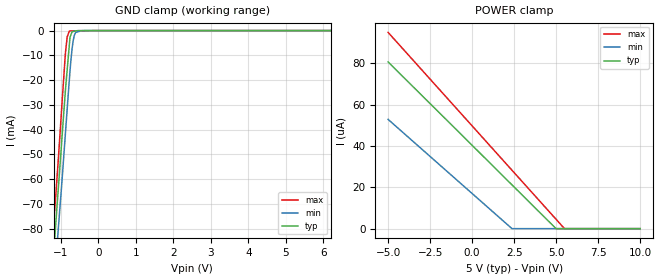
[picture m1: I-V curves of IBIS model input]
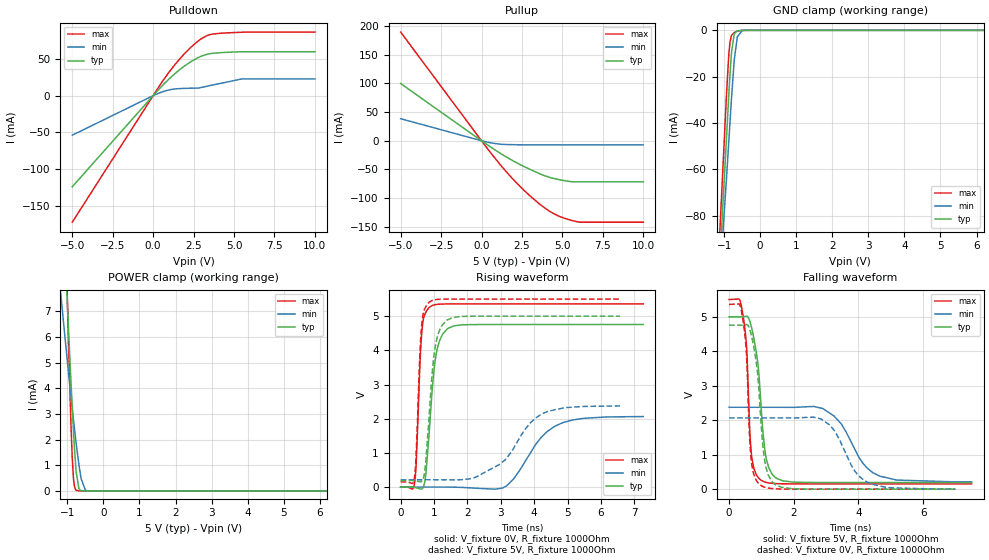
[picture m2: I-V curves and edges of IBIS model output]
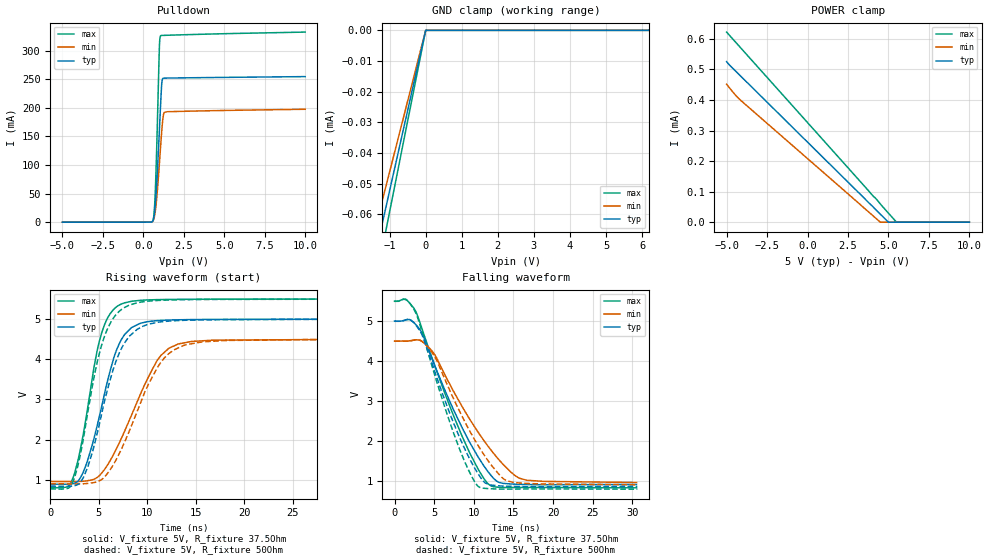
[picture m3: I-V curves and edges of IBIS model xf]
|Texas Instruments Incorporated
| ControlNet(TM) Transceiver
| Marketing part#   Digital Voltage Range   Package-type   #pins
| SN65HVD61D   2.375V-5.5V   SOIC   14
| SN65HVD61DG4   2.375V-5.5V   SOIC   14
| SN65HVD61DR   2.375V-5.5V   SOIC   14
| SN65HVD61DRG4   2.375V-5.5V   SOIC   14
[IBIS Ver]   4.1
[File name]   sn65hvd61.ibs
[File Rev]   1.0
[Date]   6/26/2013
[Source]
| Texas Instruments Incorporated.
| Analog-eLab Design Center, HPA
| 12500 TI Blvd
| Dallas, TX -75243
[Notes]   Revision History:
| Rev 1.0: 6/26/2013
| - Initial version of the model
| - Model generated from simulations in TISPICE
| - Model matched to SPICE simulation
| - C_comp although listed in numerical order of value are
|   obtained from varying PVT conditions. For PVT conditions for
|   each specific value refer the buffer description under
|   respective [Model]. IBIS model user is responsible for using
|   appropriate C_comp to simulate for Signal Integrity.
|*  EXCEPTION   *
|*  - For model input,There will be a leakage current in the power clamp I-V  *
|*   Table because of the pulldown R2(RES_P1H) resistance connected between  *
|*   ground and pad pin .   *
|*  - For model xf,There will be a leakage current in the power clamp I-V   *
|*   Table because of the RES_P1H resistances connected between   *
|*   ground and pad pin from the attenuation block   *
[Disclaimer]
| This model is designed as an aid for customers of Texas Instruments.
| TI and its licensors and suppliers make no warranties, either expressed
| or implied, with respect to this  model, including the warranties of
| merchantability or fitness for a particular purpose. The model is
| provided solely on an "as is" basis. The entire risk as to its quality
| and performance is with the customer.
[Copyright]
(C) Copyright 2013 Texas Instruments Incorporated.All rights reserved.
|   SN65HVD61
[Component]   SN65HVD61
[Manufacturer]   TI
[Package]   |14 SOIC  -  D package
|   typ   min   max
R_pkg   0.1052025   0.05633   0.14242
L_pkg   2.5378625nH  1.72746nH   3.46735nH
C_pkg   0.462875pF   0.35056pF   0.62881pF
[Pin]  signal_name   model_name   R_pin   L_pin   C_pin
1   RX   output   0.11216   3.36701nH  0.62881pF
2   CD   output   0.14102   2.79716nH  0.46799pF
3   VDD   power   0.06385   1.94248nH  0.40989pF
4   CHEN   input   0.09802   2.01847nH  0.35056pF
5   TX   input   0.11457   2.26018nH  0.36209pF
6   _TX   input   0.14242   2.82725nH  0.46580pF
7   TXEN   input   0.11690   3.46735nH  0.62224pF
8   SIG   nc   0.11238   3.40402nH  0.62049pF
9   DGND   gnd   0.06099   2.01080nH  0.49310pF
10   XF3   xf   0.06020   1.83802nH  0.40525pF
11   CGND   gnd   0.05087   1.61450nH  0.38992pF
12   XF1   xf   0.05633   1.72746nH  0.40026pF
13   CGND   gnd   0.06099   2.02284nH  0.49854pF
14   VCC   power   0.05843   3.02226nH  0.66420pF
| Models and submodels in the file (3): input (Input), output (3-state), xf (I/O_open_sink)
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|   input Model
[Model]   input
Model_type   Input
Vinl = 1.5
Vinh = 3.5
|   typ   min   max
|   (nom PVT)   (fast PVT)   (slow PVT)
C_comp   1.465e-12   1.413e-12   1.777e-12
[Model spec]
|subparameter
Vinl   1.5   0.7125   1.65
Vinh   3.50   1.6625   3.85
| Where nom  PVT is Nominal Process, 5V, 27C
|   Fast PVT is Strong Process,  5.5V, -30C
|   Slow PVT is Weak Process,   2.375V, 100C
[Voltage Range]   5   2.375   5.5
|Junction Temperature
[Temperature Range]   27   100   -30
[Power Clamp Reference]   5   2.375   5.5
[GND Clamp Reference]   0   0   0
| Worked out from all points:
|   GND clamp passes 1 mA (typ) near -0.72 V on its own axis
[GND Clamp]
|   Voltage   I(typ)   I(min)   I(max)
-5V       -570.9mA   -618.4mA   -543.7mA
-1.223V   -95.42mA   -107.8mA   -83.36mA
-1.171V   -84.48mA   -98.48mA   -72.9mA
-1.144V   -78.85mA   -93.5mA    -67.51mA
-1.081V   -65.58mA   -81.73mA   -53.82mA
-880mV    -23.57mA   -41.01mA   -8.722mA
-836mV    -15.92mA   -31.8mA    -2.607mA
-764.5mV  -3.497mA   -17.24mA   -153.8uA
-707.7mV  -549.9uA   -7.753mA   -142.4uA
-646mV    -261.4uA   -2.023mA   -129.9uA
-439.4mV  -4.594uA   -7.683uA   -88.38uA
10V       0A         0A         0A
[POWER Clamp]
|   Voltage   I(typ)   I(min)   I(max)
-5V       80.61uA    52.82uA    94.88uA
2.373V    21.18uA    17.01nA    28.26uA
4.995V    40.31nA    0A         4.563uA
5.495V    0A         0A         49.7nA
10V       0A         0A         0A
|   output Model
[Model]   output
Model_type   3-state
Polarity   Non-Inverting
Vmeas = 2.0
Vref = 0
Cref = 15pF
Rref = 1000
|   typ   min   max
|   (nom PVT)   (fast PVT)   (slow PVT)
C_comp   2.533e-12   2.400e-12   3.277e-12
| Where nom  PVT is Nominal Process, 5V, 27C
|   Fast PVT is Strong Process,  5.5V, -30C
|   Slow PVT is Weak Process,   2.375V, 100C
[Voltage Range]   5   2.375   5.5
|Junction Temperature
[Temperature Range]   27   100   -30
[Pullup Reference]   5   2.375   5.5
[Pulldown Reference]   0   0   0
[Power Clamp Reference]   5   2.375   5.5
[GND Clamp Reference]   0   0   0
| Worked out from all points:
|   slope of the pulldown table from 0 to 0.75 V, typ, clamps not added: 42.3 ohm
|   slope of the pullup table from 0 to 0.75 V, typ, clamps not added: 52.3 ohm
|   GND clamp passes 1 mA (typ) near -0.69 V on its own axis
|   POWER clamp passes 1 mA (typ) near -0.77 V on its own axis
|   falling waveform, V_fixture 5V, R_fixture 1000Ohm: 20-80 % time 275ps typ, 816ps min, 157ps max; typ from 5 V to 0.193 V
|   rising waveform, V_fixture 0V, R_fixture 1000Ohm: 20-80 % time 249ps typ, 920ps min, 134ps max; typ from 0 V to 4.76 V
|   rising waveform, V_fixture 5V, R_fixture 1000Ohm: 20-80 % time 242ps typ, 1.02ns min, 131ps max; typ from 0.193 V to 5 V
|   falling waveform, V_fixture 0V, R_fixture 1000Ohm: 20-80 % time 263ps typ, 697ps min, 154ps max; typ from 4.76 V to 0 V
[Pulldown]
|   Voltage   I(typ)   I(min)   I(max)
-5V       -124.3mA   -53.93mA   -172.6mA
0V        0A         0A         0A
557.5mV   13.43mA    5.13mA     18.87mA
989.8mV   22.89mA    7.871mA    32.21mA
1.617V    35.01mA    9.62mA     49.47mA
2.004V    41.48mA    9.97mA     58.84mA
2.75V     51.51mA    10.34mA    73.89mA
3.404V    56.8mA     13.24mA    82.5mA
4.202V    58.74mA    16.92mA    85.2mA
5.502V    59.92mA    22.88mA    86.51mA
10V       59.92mA    22.88mA    86.72mA
[GND Clamp]
|   Voltage   I(typ)   I(min)   I(max)
-5V       -869.5mA   -740.6mA   -996mA
-1.145V   -107.2mA   -113.8mA   -95.34mA
-935.5mV  -47.05mA   -64.31mA   -28.26mA
-875mV    -29.39mA   -49.25mA   -11.67mA
-865mV    -26.58mA   -46.74mA   -9.576mA
-836.5mV  -18.97mA   -39.62mA   -5.105mA
-792.5mV  -9.229mA   -28.85mA   -2.14mA
-715mV    -1.413mA   -12.29mA   -929.1uA
-632.4mV  -210.3uA   -2.765mA   -373uA
-500mV    -7.452uA   -137.4uA   -26.2uA
-375.9mV  -165.6nA   -7.725uA   -510.1nA
10V       0A         0A         0A
[Pullup]
|   Voltage   I(typ)   I(min)   I(max)
-5V       99.82mA    38.45mA    189.5mA
0V        0A         0A         0A
697.6mV   -13.38mA   -4.226mA   -25.64mA
1.605V    -29.37mA   -6.596mA   -56.31mA
2.381V    -41.42mA   -6.991mA   -79.63mA
3.692V    -58.6mA    -7.139mA   -112.5mA
4.29V     -64.44mA   -7.139mA   -124.3mA
4.806V    -67.79mA   -7.139mA   -131.7mA
5.5V      -71.17mA   -7.139mA   -138.3mA
6.061V    -71.58mA   -7.139mA   -141.9mA
10V       -71.58mA   -7.139mA   -141.9mA
[POWER Clamp]
|   Voltage   I(typ)   I(min)   I(max)
-5V       144.5mA    65.18mA    243.7mA
-1.315V   17.65mA    9.659mA    25.67mA
-1.15V    12.15mA    7.204mA    15.93mA
-1.008V   7.54mA     5.164mA    7.89mA
-902.5mV  4.327mA    3.722mA    2.689mA
-864mV    3.232mA    3.213mA    1.27mA
-805mV    1.721mA    2.457mA    187.1uA
-754mV    718.4uA    1.836mA    22.06uA
-680mV    82.57uA    1.021mA    1.038uA
-618.1mV  8.277uA    474.2uA    87.89nA
-442.4mV  0A         5.444uA    0A
10V       0A         0A         0A
[Ramp]
R_load = 1000
|   typ   min   max
dV/dt_r   2.85414/2.46472e-10   1.23967/9.10375e-10   3.21465/1.33896e-10
dV/dt_f   2.88408/2.73849e-10   1.29658/8.04689e-10   3.20839/1.56294e-10
[Falling Waveform]
V_fixture = 5V
V_fixture_min = 2.375V
V_fixture_max = 5.5V
R_fixture = 1000Ohm
|   Time   V(typ)   V(min)   V(max)
0s        5V         2.375V     5.5V
432ps     4.998V     2.375V     5.048V
544ps     5.019V     2.375V     4.099V
688ps     4.721V     2.375V     1.06V
970ps     2.707V     2.375V     275mV
1.156ns   864.2mV    2.375V     194.9mV
1.65ns    244.4mV    2.374V     155.6mV
3.248ns   193.2mV    2.12V      152.7mV
4.652ns   193.2mV    378.9mV    152.7mV
7.5ns     193.2mV    214mV      152.7mV
[Rising Waveform]
V_fixture = 0V
V_fixture_min = 0V
V_fixture_max = 0V
R_fixture = 1000Ohm
|   Time   V(typ)   V(min)   V(max)
0s        604.5pV    1.137nV    508.5pV
412ps     -11.05mV   -93.95uV   90.08mV
632ps     -55.19mV   141.1uV    4.515V
738ps     250.1mV    416.5uV    5.084V
862ps     1.709V     664.5uV    5.26V
1.07ns    3.923V     850.7uV    5.342V
1.408ns   4.637V     -444uV     5.357V
3.18ns    4.757V     40.35mV    5.358V
4.84ns    4.757V     1.88V      5.358V
7.264ns   4.757V     2.064V     5.358V
[Rising Waveform]
V_fixture = 5V
V_fixture_min = 2.375V
V_fixture_max = 5.5V
R_fixture = 1000Ohm
|   Time   V(typ)   V(min)   V(max)
0s        193.2mV    214mV      152.7mV
406ps     183.5mV    214mV      227.6mV
624ps     163.1mV    214.2mV    4.666V
726ps     493.6mV    214.4mV    5.223V
852ps     2.063V     214.4mV    5.403V
1.046ns   4.167V     213.9mV    5.483V
1.378ns   4.881V     211.9mV    5.499V
2.94ns    5V         650.6mV    5.5V
4.422ns   5V         2.221V     5.5V
6.57ns    5V         2.373V     5.5V
[Falling Waveform]
V_fixture = 0V
V_fixture_min = 0V
V_fixture_max = 0V
R_fixture = 1000Ohm
|   Time   V(typ)   V(min)   V(max)
0s        4.757V     2.066V     5.358V
428ps     4.755V     2.066V     4.92V
536ps     4.775V     2.066V     3.984V
680ps     4.502V     2.066V     901.3mV
962ps     2.315V     2.066V     124.1mV
1.136ns   654.5mV    2.066V     47.22mV
1.628ns   53.12mV    2.065V     3.601mV
3.112ns   52.29uV    1.862V     -6.142uV
4.374ns   -3.292uV   154.7mV    450.8nV
7ns       395.4pV    1.275nV    100.5pV
|   xf Model
[Model]   xf
Model_type   I/O_open_sink
Polarity   Inverting
Enable   Active-High
Vinl=1.5
Vinh=3.5
Vmeas = 2.5
Vref = 5
Cref = 15pF
Rref = 37.5
|   typ   min   max
|   (nom PVT)   (fast PVT)   (slow PVT)
C_comp   2.264e-11   2.099e-11   2.458e-11
[Model spec]
|subparameter
Vinl   1.5   1.35   1.65
Vinh   3.50   3.15   3.85
| Where nom  PVT is Nominal Process, 5V, 27C
|   Fast PVT is Strong Process,  5.5V, -30C
|   Slow PVT is Weak Process,   4.5V, 100C
[Voltage Range]   5   4.5   5.5
|Junction Temperature
[Temperature Range]   27   100   -30
[Pullup Reference]   5   4.5   5.5
[Pulldown Reference]   0   0   0
[Power Clamp Reference]   5   4.5   5.5
[GND Clamp Reference]   0   0   0
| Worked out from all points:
|   slope of the pulldown table from 0 to 0.75 V, typ, clamps not added: 21.4 ohm
|   falling waveform, V_fixture 5V, R_fixture 37.5Ohm: 20-80 % time 5.67ns typ, 6.57ns min, 5.46ns max; typ from 4.99 V to 0.908 V
|   rising waveform, V_fixture 5V, R_fixture 37.5Ohm: 20-80 % time 2.62ns typ, 4.01ns min, 2.1ns max; typ from 0.905 V to 4.99 V
|   falling waveform, V_fixture 5V, R_fixture 50Ohm: 20-80 % time 4.79ns typ, 5.55ns min, 4.61ns max; typ from 4.99 V to 0.858 V
|   rising waveform, V_fixture 5V, R_fixture 50Ohm: 20-80 % time 2.81ns typ, 3.97ns min, 2.39ns max; typ from 0.856 V to 4.99 V
[Pulldown]
|   Voltage   I(typ)   I(min)   I(max)
-5V       -50.3pA    -5.4pA     -101.8pA
566.5mV   1.445mA    1.464mA    1.227mA
661mV     10.26mA    6.97mA     15.21mA
725.5mV   26.45mA    16.5mA     45.69mA
805mV     58.08mA    35.69mA    109.7mA
994mV     162.4mA    103.3mA    307.9mA
1.034V    186.1mA    119.2mA    323.5mA
1.09V     219.3mA    141.7mA    326.3mA
1.16V     248.1mA    167.3mA    326.6mA
1.225V    251.6mA    184.9mA    326.7mA
1.3V      252mA      192.1mA    326.7mA
10V       254.6mA    197.5mA    332.4mA
[GND Clamp]
|   Voltage   I(typ)   I(min)   I(max)
-5V       -261.6uA   -230.7uA   -295.9uA
-1.472V   -77.01uA   -67.94uA   -87.11uA
-820mV    -42.9uA    -37.85uA   -48.52uA
-84.44fV  0A         -21.89nA   -28.29nA
10V       0A         0A         0A
[POWER Clamp]
|   Voltage   I(typ)   I(min)   I(max)
-5V       525.6uA    451.4uA    622.2uA
-4.402V   492.4uA    413.2uA    586.7uA
-4.091V   476.1uA    397.1uA    568.3uA
4.5V      26.18uA    23.14nA    59.7uA
4.995V    261.5nA    0A         29.88uA
5.5V      0A         0A         29.54nA
10V       0A         0A         0A
[Ramp]
R_load = 37.5
|   typ   min   max
dV/dt_r   2.45114/2.60432e-09   2.11333/4.01179e-09   2.80026/2.09082e-09
dV/dt_f   2.45171/5.6729e-09   2.11213/6.53226e-09   2.80004/5.46525e-09
[Falling Waveform]
V_fixture = 5V
V_fixture_min = 4.5V
V_fixture_max = 5.5V
R_fixture = 37.5Ohm
|   Time   V(typ)   V(min)   V(max)
0s        4.989V     4.491V     5.487V
1.6ns     5.029V     4.492V     5.504V
2.6ns     4.921V     4.518V     5.262V
3.225ns   4.772V     4.508V     4.944V
5.1ns     3.866V     4.143V     3.864V
8.55ns    2.317V     2.847V     2.104V
11.85ns   1.214V     1.85V      915.3mV
13.22ns   957.5mV    1.514V     835.4mV
16.67ns   907.2mV    1.013V     832.7mV
30.52ns   908.2mV    956.5mV    824.3mV
[Rising Waveform]
V_fixture = 5V
V_fixture_min = 4.5V
V_fixture_max = 5.5V
R_fixture = 37.5Ohm
|   Time   V(typ)   V(min)   V(max)
0s        904.9mV    969.9mV    820.7mV
2.075ns   905.9mV    968.4mV    902.9mV
3.275ns   1.138V     974.3mV    1.975V
5.075ns   2.593V     1.118V     4.454V
5.95ns    3.501V     1.394V     5.035V
7.075ns   4.361V     1.903V     5.334V
8.425ns   4.786V     2.637V     5.433V
11.07ns   4.953V     3.986V     5.473V
13.2ns    4.974V     4.375V     5.48V
31.63ns   4.989V     4.489V     5.487V
[Falling Waveform]
V_fixture = 5V
V_fixture_min = 4.5V
V_fixture_max = 5.5V
R_fixture = 50Ohm
|   Time   V(typ)   V(min)   V(max)
0s        4.986V     4.488V     5.483V
1.6ns     5.032V     4.489V     5.511V
2.675ns   4.896V     4.522V     5.199V
3.425ns   4.667V     4.49V      4.75V
5.05ns    3.744V     4.108V     3.658V
7.45ns    2.444V     3.05V      2.196V
10.5ns    1.19V      1.896V     868.9mV
11.48ns   940.5mV    1.594V     809.1mV
14.13ns   865.2mV    1.002V     791.6mV
30.62ns   857.7mV    899.8mV    790.3mV
[Rising Waveform]
V_fixture = 5V
V_fixture_min = 4.5V
V_fixture_max = 5.5V
R_fixture = 50Ohm
|   Time   V(typ)   V(min)   V(max)
0s        855.7mV    911.3mV    788.2mV
2.125ns   854.1mV    909.2mV    854.2mV
3.375ns   1.051V     913.1mV    1.978V
4.625ns   1.951V     949.3mV    3.684V
5.475ns   2.838V     1.054V     4.481V
6.825ns   3.976V     1.523V     5.114V
8.2ns     4.576V     2.247V     5.34V
11.1ns    4.912V     3.81V      5.453V
14.02ns   4.963V     4.357V     5.472V
50ns      4.987V     4.49V      5.484V
